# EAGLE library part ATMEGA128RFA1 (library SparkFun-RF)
Atmel ATmega128RFA1 8-Bit AVR Microcontroller w/ Low-Power 2.4GHz RF Transceiver The ATmega128RFA1 is a low-power CMOS 8-bit microcontroller based on the AVR enhanced RISC architecture combined with a high data rate transceiver for the 2.4 GHz ISM band. By executing powerful instructions in a single clock cycle, the device achieves throughputs approaching 1 MIPS per MHz allowing the system designer to optimize power consumption versus processing speed. The radio transceiver provides high data rates from 250 kb/s up to 2 Mb/s, frame handling, outstanding receiver sensitivity and high transmit output power enabling a very robust wireless communication. Datasheet SparkFun ATmega128RFA1 Development Board
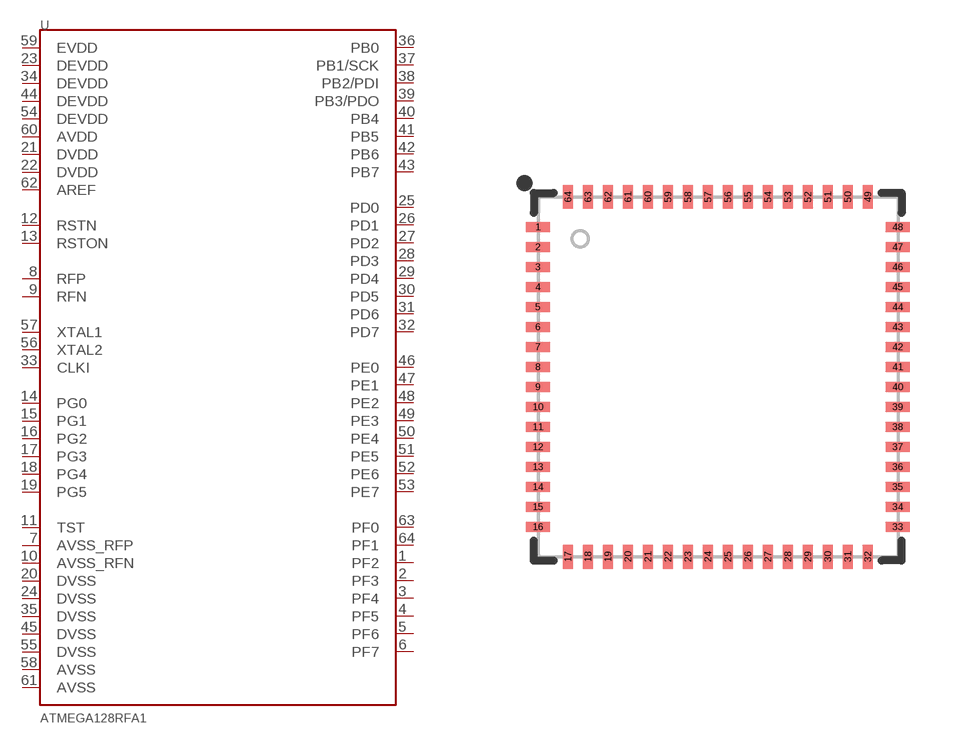
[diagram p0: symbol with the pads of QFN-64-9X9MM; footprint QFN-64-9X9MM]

Designator prefix U

## ATMEGA128RFA1 (PROD_ID: IC-09639)  [QFN-64-9X9MM]
1  PF2
2  PF3
3  PF4
4  PF5
5  PF6
6  PF7
7  AVSS_RFP
8  RFP
9  RFN
10  AVSS_RFN
11  TST
12  RSTN
13  RSTON
14  PG0
15  PG1
16  PG2
17  PG3
18  PG4
19  PG5
20  DVSS
21  DVDD
22  DVDD
23  DEVDD
24  DVSS
25  PD0
26  PD1
27  PD2
28  PD3
29  PD4
30  PD5
31  PD6
32  PD7
33  CLKI
34  DEVDD
35  DVSS
36  PB0
37  PB1/SCK
38  PB2/PDI
39  PB3/PDO
40  PB4
41  PB5
42  PB6
43  PB7
44  DEVDD
45  DVSS
46  PE0
47  PE1
48  PE2
49  PE3
50  PE4
51  PE5
52  PE6
53  PE7
54  DEVDD
55  DVSS
56  XTAL2
57  XTAL1
58  AVSS
59  EVDD
60  AVDD
61  AVSS
62  AREF
63  PF0
64  PF1

## Footprint QFN-64-9X9MM (pad centres in mm)
64-pin QFN 9x9mm, 0.5mm pitch Package used by ATmega128RFA1 Example Datasheet
smd 0.6 x 0.25: 1 -4.5,3.75; 2 -4.5,3.25; 3 -4.5,2.75; 4 -4.5,2.25; 5 -4.5,1.75; 6 -4.5,1.25; 7 -4.5,0.75; 8 -4.5,0.25; 9 -4.5,-0.25; 10 -4.5,-0.75; 11 -4.5,-1.25; 12 -4.5,-1.75; 13 -4.5,-2.25; 14 -4.5,-2.75; 15 -4.5,-3.25; 16 -4.5,-3.75; 33 4.5,-3.75; 34 4.5,-3.25; 35 4.5,-2.75; 36 4.5,-2.25; 37 4.5,-1.75; 38 4.5,-1.25; 39 4.5,-0.75; 40 4.5,-0.25; 41 4.5,0.25; 42 4.5,0.75; 43 4.5,1.25; 44 4.5,1.75; 45 4.5,2.25; 46 4.5,2.75; 47 4.5,3.25; 48 4.5,3.75
smd 0.25 x 0.6: 17 -3.75,-4.5; 18 -3.25,-4.5; 19 -2.75,-4.5; 20 -2.25,-4.5; 21 -1.75,-4.5; 22 -1.25,-4.5; 23 -0.75,-4.5; 24 -0.25,-4.5; 25 0.25,-4.5; 26 0.75,-4.5; 27 1.25,-4.5; 28 1.75,-4.5; 29 2.25,-4.5; 30 2.75,-4.5; 31 3.25,-4.5; 32 3.75,-4.5; 49 3.75,4.5; 50 3.25,4.5; 51 2.75,4.5; 52 2.25,4.5; 53 1.75,4.5; 54 1.25,4.5; 55 0.75,4.5; 56 0.25,4.5; 57 -0.25,4.5; 58 -0.75,4.5; 59 -1.25,4.5; 60 -1.75,4.5; 61 -2.25,4.5; 62 -2.75,4.5; 63 -3.25,4.5; 64 -3.75,4.5

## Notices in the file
Licensing: Creative Commons ShareAlike 4.0 International - https://creativecommons.org/licenses/by-sa/4.0
© 2015 RF Digital Corporation
